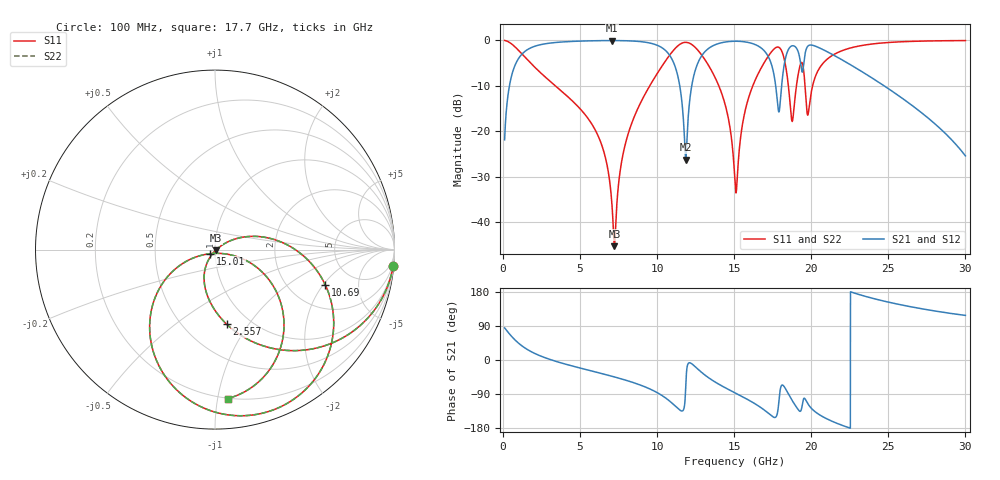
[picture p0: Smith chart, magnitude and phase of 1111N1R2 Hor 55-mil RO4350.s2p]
# GHz S MA R 50
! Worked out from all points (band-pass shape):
!   3201 points, 100 MHz to 30 GHz, reference 50 ohm
!   highest |S21| = -0.05 dB at 7.052 GHz (marker M1); lowest = -26.3 dB at 11.85 GHz (marker M2)
!   |S21| within 3 dB of the highest: 1.221 GHz to 10.76 GHz (9.537 GHz wide, 159 % of centre); 12.96 GHz to 17.12 GHz (4.156 GHz wide, 27.6 % of centre)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
!   lowest |S11| = -45.3 dB at 7.229 GHz (marker M3), VSWR 1.01, Z = 50.4 - j0.367 ohm
!   |S11| at or under -10 dB: 3.386 GHz to 9.521 GHz (6.135 GHz wide, 95.1 % of centre); 14 GHz to 16.21 GHz (2.209 GHz wide, 14.6 % of centre); 18.51 GHz to 19.04 GHz (524.3 MHz wide, 2.79 % of centre)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
!   |S22| runs from -45.3 to 0.0 dB; largest |S21 - S12| = 0
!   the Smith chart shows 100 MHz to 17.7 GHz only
!   S11 on the Smith chart (normalised r, x): 100 MHz: 1, -22; 2.557 GHz: 0.79, -0.79; 10.69 GHz: 3.13, -2.08; 15.01 GHz: 0.95, -0.04; 17.7 GHz: 0.20, -1.07
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0.1  0.9967 -5.3  0.08037 84.7  0.08037 84.7  0.9967 -5.3
0.8194687  0.8331 -38.8  0.5523 51.2  0.5523 51.2  0.8331 -38.8
2.557406  0.4204 -81.1  0.905 8.6  0.905 8.6  0.4204 -81.1
5.089563  0.1696 -111.0  0.9816 -22.2  0.9816 -22.2  0.1696 -111.0
7.05175  0.0167 -114.7  0.9939 -42.7  0.9939 -42.7  0.0167 -114.7
7.229281  0.005423 -42.2  0.9938 -44.7  0.9938 -44.7  0.005423 -42.2
8.051531  0.08576 31.0  0.9885 -54.4  0.9885 -54.4  0.08576 31.0
10.06978  0.4494 -0.2  0.8725 -87.7  0.8725 -87.7  0.4494 -0.2
10.68647  0.644 -17.6  0.7286 -104.5  0.7286 -104.5  0.644 -17.6
11.85444  0.9503 -70.9  0.04841 -68.4  0.04841 -68.4  0.9503 -70.9
12.72341  0.7487 -112.6  0.6041 -27.1  0.6041 -27.1  0.7487 -112.6
14.33987  0.2163 -155.7  0.953 -71.6  0.953 -71.6  0.2163 -155.7
15.01262  0.03499 -139.4  0.9772 -85.9  0.9772 -85.9  0.03499 -139.4
15.05  0.02745 -127.2  0.9774 -86.7  0.9774 -86.7  0.02745 -127.2
15.97503  0.2457 -22.6  0.9424 -106.6  0.9424 -106.6  0.2457 -22.6
17.70362  0.8327 -85.2  0.3025 -150.4  0.3025 -150.4  0.8327 -85.2
18.22687  0.6403 -130.9  0.5182 -69.5  0.5182 -69.5  0.6403 -130.9
18.75013  0.1284 -106.2  0.8696 -106.3  0.8696 -106.3  0.1284 -106.2
19.32009  0.5588 -84.9  0.539 -134.2  0.539 -134.2  0.5588 -84.9
20.03956  0.2908 -53.3  0.8855 -129.0  0.8855 -129.0  0.2908 -53.3
25.01978  0.947 -118.7  0.2923 152.5  0.2923 152.5  0.947 -118.7
30  0.9934 -154.4  0.05351 117.7  0.05351 117.7  0.9934 -154.4
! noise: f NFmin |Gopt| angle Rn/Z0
0.1  0.002637  0.9391  2.369  0.009657
3.417  0.01284  0.5795  24.57  0.005322
6.743  0.02452  0.573  42.23  0.009147
10.06  0.06246  0.7327  59.47  0.03542
13.39  0.09391  0.7639  80.3  0.04781
16.7  0.1174  0.7669  94.97  0.0478
20.03  0.1639  0.7971  112.1  0.05364
23.35  0.1449  0.76  123.5  0.0292
26.67  0.2619  0.8604  138.9  0.05158
30  0.7657  0.9514  155.6  0.1606
